| IBIS file stm32l0_51_52_53_62_63_tfbga64.ibs
| Created by s2ibis version 1.1 (customized version)
| North Carolina State University, ERL, 2006
[IBIS ver] 4.2
[File name] stm32l0_51_52_53_62_63_tfbga64.ibs
[File Rev] 1.0
[Date]  15-10-2014
[Source] Data Created at STMicroelectronics
[Notes]  File originated from ELDO simulations.
[Disclaimer]  This information is for modeling purpose only and is
   not guaranted. The information is subject to change without
   notice.
[Copyright] Copyright 2016 STMicroelectronics Inc.
|   Component stm32l0_51_52_53_62_63_tfbga64
[Component] stm32l0_51_52_53_62_63_tfbga64
[Manufacturer] STMicroelectronics
[Package]
| variable   typ   min   max
R_pkg   0.0   0.0   0.0
L_pkg   0.0H   0.0H   0.0H
C_pkg   0.0F   0.0F   0.0F
[Pin]  signal_name   model_name   R_pin   L_pin   C_pin
B2 VLCD POWER
A2 PC13 io8p_wsudq_ls_ft_v33
A1 PC14-OSC32_IN io8p_wsudq_ls_ft_v33
B1 PC15-OSC32_OUT io8p_sudq_ls_tc_esdft
C1 PH0-OSC_IN io8p_sudq_ls_tc_esdft
D1 PH1-OSC_OUT io8p_sudq_ls_tc_esdft
E1 NRST ioreset_tc_v33_esdft
E3 PC0 io8p_wsudq_lcd4_ls_ft
E2 PC1 io8p_wsudq_lcd4_ls_ft
F2 PC2 io8p_wsudq_lcd4_ls_ft
F1 VSSA GND
G1 VREF+ POWER
H1 VDDA POWER
G2 PA0 io8p_wsudq_ls_ft_v33
H2 PA1 io8p_wsudq_lcd4_ls_ft
F3 PA2 io8p_wsudq_lcd4_ls_ft
G3 PA3 io8p_wsudq_lcd4_ls_ft
C2 VSS GND
D2 VDD POWER
H3 PA4 io8p_wsudq_i2cin_ls_ft
F4 PA5 io8p_wsudq_i2cin_ls_ft
G4 PA6 io8p_wsudq_lcd4_ls_ft
H4 PA7 io8p_wsudq_lcd4_ls_ft
H5 PC4 io8p_wsudq_lcd4_ls_ft
H6 PC5 io8p_wsudq_lcd4_ls_ft
F5 PB0 io8p_wsudq_lcd4_ls_ft
G5 PB1 io8p_wsudq_lcd4_ls_ft
G6 PB2 io8p_wsudq_lcd4_ls_ft
G7 PB10 io8p_sudq_lcd4_i2cin_ls_ft
H7 PB11 io8p_sudq_lcd4_i2cin_ls_ft
D6 VSS GND
E5 VDD POWER
H8 PB12 io8p_wsudq_lcd4_ls_ft
G8 PB13 io8p_sudq_lcd4_i2cin_ls_ft
F8 PB14 io8p_sudq_lcd4_i2cin_ls_ft
F7 PB15 io8p_wsudq_lcd4_ls_ft
F6 PC6 io8p_wsudq_lcd4_ls_ft
E7 PC7 io8p_wsudq_lcd4_ls_ft
E8 PC8 io8p_wsudq_lcd4_ls_ft
D8 PC9 io8p_wsudq_lcd4_ls_ft
D7 PA8 io8p_wsudq_lcd4_ls_ft
C7 PA9 io8p_wsudq_lcd4_ls_ft
C6 PA10 io8p_wsudq_lcd4_ls_ft
C8 PA11 io8usb_ls_ft
B8 PA12 io8usb_ls_ft
A8 PA13 io8p_sudq_ls_ft
D5 VSS GND
E6 VDD_USB POWER
A7 PA14 io8p_sudq_ls_ft
A6 PA15 io8p_wsudq_lcd4_ls_ft
B7 PC10 io8p_wsudq_lcd4_ls_ft
B6 PC11 io8p_wsudq_lcd4_ls_ft
C5 PC12 io8p_wsudq_lcd4_ls_ft
B5 PD2 io8p_wsudq_lcd4_ls_ft
A5 PB3 io8p_wsudq_lcd4_ls_ft
A4 PB4 io8p_wsudq_lcd4_ls_ft
C4 PB5 io8p_wsudq_lcd4_ls_ft
D3 PB6 io8p_wsudq_i2cin_ls_ft
C3 PB7 io8p_wsudq_i2cin_ls_ft
B4 BOOT0 vpp_test_hv
B3 PB8 io8p_sudq_lcd4_i2cin_ls_ft
A3 PB9 io8p_sudq_lcd4_i2cin_ls_ft
D4 VSS_3 GND
E4 VDD_3 POWER
[Model Selector] io8p_sudq_ls_ft
io8p00_sudq_ls_ft_pd_lv  "SPEED00 1P8V, PD=40kOhm"
io8p00_sudq_ls_ft_pu_lv  "SPEED00 1P8V, PU=40kOhm"
io8p00_sudq_ls_ft_lv  "SPEED00 1P8V"
io8p01_sudq_ls_ft_pd_lv  "SPEED01 1P8V, PD=40kOhm"
io8p01_sudq_ls_ft_pu_lv  "SPEED01 1P8V, PU=40kOhm"
io8p01_sudq_ls_ft_lv  "SPEED01 1P8V"
io8p10_sudq_ls_ft_pd_lv  "SPEED10 1P8V, PD=40kOhm"
io8p10_sudq_ls_ft_pu_lv  "SPEED10 1P8V, PU=40kOhm"
io8p10_sudq_ls_ft_lv  "SPEED10 1P8V"
io8p11_sudq_ls_ft_pd_lv  "SPEED11 1P8V, PD=40kOhm"
io8p11_sudq_ls_ft_pu_lv  "SPEED11 1P8V, PU=40kOhm"
io8p11_sudq_ls_ft_lv  "SPEED11 1P8V"
io8p00_sudq_ls_ft_pd  "SPEED00, PD=40kOhm"
io8p00_sudq_ls_ft_pu  "SPEED00, PU=40kOhm"
io8p00_sudq_ls_ft  "SPEED00"
io8p01_sudq_ls_ft_pd  "SPEED01, PD=40kOhm"
io8p01_sudq_ls_ft_pu  "SPEED01, PU=40kOhm"
io8p01_sudq_ls_ft  "SPEED01"
io8p10_sudq_ls_ft_pd  "SPEED10, PD=40kOhm"
io8p10_sudq_ls_ft_pu  "SPEED10, PU=40kOhm"
io8p10_sudq_ls_ft  "SPEED10"
io8p11_sudq_ls_ft_pd  "SPEED11, PD=40kOhm"
io8p11_sudq_ls_ft_pu  "SPEED11, PU=40kOhm"
io8p11_sudq_ls_ft  "SPEED11"
[Model Selector] io8p_sudq_ls_tc_esdft
io8p00_sudq_ls_tc_esdft_pd_lv  "SPEED00 1P8V, PD=40kOhm"
io8p00_sudq_ls_tc_esdft_pu_lv  "SPEED00 1P8V, PU=40kOhm"
io8p00_sudq_ls_tc_esdft_lv  "SPEED00 1P8V"
io8p01_sudq_ls_tc_esdft_pd_lv  "SPEED01 1P8V, PD=40kOhm"
io8p01_sudq_ls_tc_esdft_pu_lv  "SPEED01 1P8V, PU=40kOhm"
io8p01_sudq_ls_tc_esdft_lv  "SPEED01 1P8V"
io8p10_sudq_ls_tc_esdft_pd_lv  "SPEED10 1P8V, PD=40kOhm"
io8p10_sudq_ls_tc_esdft_pu_lv  "SPEED10 1P8V, PU=40kOhm"
io8p10_sudq_ls_tc_esdft_lv  "SPEED10 1P8V"
io8p11_sudq_ls_tc_esdft_pd_lv  "SPEED11 1P8V, PD=40kOhm"
io8p11_sudq_ls_tc_esdft_pu_lv  "SPEED11 1P8V, PU=40kOhm"
io8p11_sudq_ls_tc_esdft_lv  "SPEED11 1P8V"
io8p00_sudq_ls_tc_esdft_pd  "SPEED00, PD=40kOhm"
io8p00_sudq_ls_tc_esdft_pu  "SPEED00, PU=40kOhm"
io8p00_sudq_ls_tc_esdft  "SPEED00"
io8p01_sudq_ls_tc_esdft_pd  "SPEED01, PD=40kOhm"
io8p01_sudq_ls_tc_esdft_pu  "SPEED01, PU=40kOhm"
io8p01_sudq_ls_tc_esdft  "SPEED01"
io8p10_sudq_ls_tc_esdft_pd  "SPEED10, PD=40kOhm"
io8p10_sudq_ls_tc_esdft_pu  "SPEED10, PU=40kOhm"
io8p10_sudq_ls_tc_esdft  "SPEED10"
io8p11_sudq_ls_tc_esdft_pd  "SPEED11, PD=40kOhm"
io8p11_sudq_ls_tc_esdft_pu  "SPEED11, PU=40kOhm"
io8p11_sudq_ls_tc_esdft  "SPEED11"
[Model Selector] io8p_wsudq_i2cin_ls_ft
io8p00_wsudq_i2cin_ls_ft_pd_lv  "SPEED00 1P8V, PD=40kOhm"
io8p00_wsudq_i2cin_ls_ft_pu_lv  "SPEED00 1P8V, PU=40kOhm"
io8p00_wsudq_i2cin_ls_ft_lv  "SPEED00 1P8V"
io8p01_wsudq_i2cin_ls_ft_pd_lv  "SPEED01 1P8V, PD=40kOhm"
io8p01_wsudq_i2cin_ls_ft_pu_lv  "SPEED01 1P8V, PU=40kOhm"
io8p01_wsudq_i2cin_ls_ft_lv  "SPEED01 1P8V"
io8p10_wsudq_i2cin_ls_ft_pd_lv  "SPEED10 1P8V, PD=40kOhm"
io8p10_wsudq_i2cin_ls_ft_pu_lv  "SPEED10 1P8V, PU=40kOhm"
io8p10_wsudq_i2cin_ls_ft_lv  "SPEED10 1P8V"
io8p11_wsudq_i2cin_ls_ft_pd_lv  "SPEED11 1P8V, PD=40kOhm"
io8p11_wsudq_i2cin_ls_ft_pu_lv  "SPEED11 1P8V, PU=40kOhm"
io8p11_wsudq_i2cin_ls_ft_lv  "SPEED11 1P8V"
io8p00_wsudq_i2cin_ls_ft_pd  "SPEED00, PD=40kOhm"
io8p00_wsudq_i2cin_ls_ft_pu  "SPEED00, PU=40kOhm"
io8p00_wsudq_i2cin_ls_ft  "SPEED00"
io8p01_wsudq_i2cin_ls_ft_pd  "SPEED01, PD=40kOhm"
io8p01_wsudq_i2cin_ls_ft_pu  "SPEED01, PU=40kOhm"
io8p01_wsudq_i2cin_ls_ft  "SPEED01"
io8p10_wsudq_i2cin_ls_ft_pd  "SPEED10, PD=40kOhm"
io8p10_wsudq_i2cin_ls_ft_pu  "SPEED10, PU=40kOhm"
io8p10_wsudq_i2cin_ls_ft  "SPEED10"
io8p11_wsudq_i2cin_ls_ft_pd  "SPEED11, PD=40kOhm"
io8p11_wsudq_i2cin_ls_ft_pu  "SPEED11, PU=40kOhm"
io8p11_wsudq_i2cin_ls_ft  "SPEED11"
[Model Selector] io8p_wsudq_lcd4_ls_ft
io8p00_wsudq_lcd4_ls_ft_pd_lv  "SPEED00 1P8V, PD=40kOhm"
io8p00_wsudq_lcd4_ls_ft_pu_lv  "SPEED00 1P8V, PU=40kOhm"
io8p00_wsudq_lcd4_ls_ft_lv  "SPEED00 1P8V"
io8p01_wsudq_lcd4_ls_ft_pd_lv  "SPEED01 1P8V, PD=40kOhm"
io8p01_wsudq_lcd4_ls_ft_pu_lv  "SPEED01 1P8V, PU=40kOhm"
io8p01_wsudq_lcd4_ls_ft_lv  "SPEED01 1P8V"
io8p10_wsudq_lcd4_ls_ft_pd_lv  "SPEED10 1P8V, PD=40kOhm"
io8p10_wsudq_lcd4_ls_ft_pu_lv  "SPEED10 1P8V, PU=40kOhm"
io8p10_wsudq_lcd4_ls_ft_lv  "SPEED10 1P8V"
io8p11_wsudq_lcd4_ls_ft_pd_lv  "SPEED11 1P8V, PD=40kOhm"
io8p11_wsudq_lcd4_ls_ft_pu_lv  "SPEED11 1P8V, PU=40kOhm"
io8p11_wsudq_lcd4_ls_ft_lv  "SPEED11 1P8V"
io8p00_wsudq_lcd4_ls_ft_pd  "SPEED00, PD=40kOhm"
io8p00_wsudq_lcd4_ls_ft_pu  "SPEED00, PU=40kOhm"
io8p00_wsudq_lcd4_ls_ft  "SPEED00"
io8p01_wsudq_lcd4_ls_ft_pd  "SPEED01, PD=40kOhm"
io8p01_wsudq_lcd4_ls_ft_pu  "SPEED01, PU=40kOhm"
io8p01_wsudq_lcd4_ls_ft  "SPEED01"
io8p10_wsudq_lcd4_ls_ft_pd  "SPEED10, PD=40kOhm"
io8p10_wsudq_lcd4_ls_ft_pu  "SPEED10, PU=40kOhm"
io8p10_wsudq_lcd4_ls_ft  "SPEED10"
io8p11_wsudq_lcd4_ls_ft_pd  "SPEED11, PD=40kOhm"
io8p11_wsudq_lcd4_ls_ft_pu  "SPEED11, PU=40kOhm"
io8p11_wsudq_lcd4_ls_ft  "SPEED11"
[Model Selector] io8p_wsudq_ls_ft_v33
io8p00_wsudq_ls_ft_v33_pd_lv  "SPEED00 1P8V, PD=40kOhm"
io8p00_wsudq_ls_ft_v33_pu_lv  "SPEED00 1P8V, PU=40kOhm"
io8p00_wsudq_ls_ft_v33_lv  "SPEED00 1P8V"
io8p01_wsudq_ls_ft_v33_pd_lv  "SPEED01 1P8V, PD=40kOhm"
io8p01_wsudq_ls_ft_v33_pu_lv  "SPEED01 1P8V, PU=40kOhm"
io8p01_wsudq_ls_ft_v33_lv  "SPEED01 1P8V"
io8p10_wsudq_ls_ft_v33_pd_lv  "SPEED10 1P8V, PD=40kOhm"
io8p10_wsudq_ls_ft_v33_pu_lv  "SPEED10 1P8V, PU=40kOhm"
io8p10_wsudq_ls_ft_v33_lv  "SPEED10 1P8V"
io8p11_wsudq_ls_ft_v33_pd_lv  "SPEED11 1P8V, PD=40kOhm"
io8p11_wsudq_ls_ft_v33_pu_lv  "SPEED11 1P8V, PU=40kOhm"
io8p11_wsudq_ls_ft_v33_lv  "SPEED11 1P8V"
io8p00_wsudq_ls_ft_v33_pd  "SPEED00, PD=40kOhm"
io8p00_wsudq_ls_ft_v33_pu  "SPEED00, PU=40kOhm"
io8p00_wsudq_ls_ft_v33  "SPEED00"
io8p01_wsudq_ls_ft_v33_pd  "SPEED01, PD=40kOhm"
io8p01_wsudq_ls_ft_v33_pu  "SPEED01, PU=40kOhm"
io8p01_wsudq_ls_ft_v33  "SPEED01"
io8p10_wsudq_ls_ft_v33_pd  "SPEED10, PD=40kOhm"
io8p10_wsudq_ls_ft_v33_pu  "SPEED10, PU=40kOhm"
io8p10_wsudq_ls_ft_v33  "SPEED10"
io8p11_wsudq_ls_ft_v33_pd  "SPEED11, PD=40kOhm"
io8p11_wsudq_ls_ft_v33_pu  "SPEED11, PU=40kOhm"
io8p11_wsudq_ls_ft_v33  "SPEED11"
[Model Selector] ioreset_tc_v33_esdft
ioreset_tc_v33_esdft_pu_lv  "IORESET 1P65V + PU=40kOhm"
ioreset_tc_v33_esdft_nopu_lv  "IORESET 1P65V"
ioreset_tc_v33_esdft_pu  "IORESET + PU=40kOhm"
ioreset_tc_v33_esdft_nopu  "IORESET"
[Model Selector] vpp_test_hv
vpp_test_hv_2p4  "Input Buffer 1P65V"
vpp_test_hv_3p3  "Input Buffer"
[Model Selector] io8usb_ls_ft
io8usb_ls_ft_dpdn_pu  "HS USB DP/DN IO + PU=1.2kOhm"
io8usb_ls_ft_dpdn  "HS USB DP/DN IO"
io8p00_ls_ft_pd_lv  "SPEED00 1P8V, PD=40kOhm"
io8p00_ls_ft_pu_lv  "SPEED00 1P8V, PU=40kOhm"
io8p00_ls_ft_lv  "SPEED00 1P8V"
io8p01_ls_ft_pd_lv  "SPEED01 1P8V, PD=40kOhm"
io8p01_ls_ft_pu_lv  "SPEED01 1P8V, PU=40kOhm"
io8p01_ls_ft_lv  "SPEED01 1P8V"
io8p10_ls_ft_pd_lv  "SPEED10 1P8V, PD=40kOhm"
io8p10_ls_ft_pu_lv  "SPEED10 1P8V, PU=40kOhm"
io8p10_ls_ft_lv  "SPEED10 1P8V"
io8p11_ls_ft_pd_lv  "SPEED11 1P8V, PD=40kOhm"
io8p11_ls_ft_pu_lv  "SPEED11 1P8V, PU=40kOhm"
io8p11_ls_ft_lv  "SPEED11 1P8V"
io8p00_ls_ft_pd  "SPEED00, PD=40kOhm"
io8p00_ls_ft_pu  "SPEED00, PU=40kOhm"
io8p00_ls_ft  "SPEED00"
io8p01_ls_ft_pd  "SPEED01, PD=40kOhm"
io8p01_ls_ft_pu  "SPEED01, PU=40kOhm"
io8p01_ls_ft  "SPEED01"
io8p10_ls_ft_pd  "SPEED10, PD=40kOhm"
io8p10_ls_ft_pu  "SPEED10, PU=40kOhm"
io8p10_ls_ft  "SPEED10"
io8p11_ls_ft_pd  "SPEED11, PD=40kOhm"
io8p11_ls_ft_pu  "SPEED11, PU=40kOhm"
io8p11_ls_ft  "SPEED11"
[Model Selector] io8p_sudq_lcd4_i2cin_ls_ft
io8p00_sudq_lcd4_i2cin_ls_ft_pd_lv  "SPEED00 1P8V, PD=40kOhm"
io8p00_sudq_lcd4_i2cin_ls_ft_pu_lv  "SPEED00 1P8V, PU=40kOhm"
io8p00_sudq_lcd4_i2cin_ls_ft_lv  "SPEED00 1P8V"
io8p01_sudq_lcd4_i2cin_ls_ft_pd_lv  "SPEED01 1P8V, PD=40kOhm"
io8p01_sudq_lcd4_i2cin_ls_ft_pu_lv  "SPEED01 1P8V, PU=40kOhm"
io8p01_sudq_lcd4_i2cin_ls_ft_lv  "SPEED01 1P8V"
io8p10_sudq_lcd4_i2cin_ls_ft_pd_lv  "SPEED10 1P8V, PD=40kOhm"
io8p10_sudq_lcd4_i2cin_ls_ft_pu_lv  "SPEED10 1P8V, PU=40kOhm"
io8p10_sudq_lcd4_i2cin_ls_ft_lv  "SPEED10 1P8V"
io8p11_sudq_lcd4_i2cin_ls_ft_pd_lv  "SPEED11 1P8V, PD=40kOhm"
io8p11_sudq_lcd4_i2cin_ls_ft_pu_lv  "SPEED11 1P8V, PU=40kOhm"
io8p11_sudq_lcd4_i2cin_ls_ft_lv  "SPEED11 1P8V"
io8p00_sudq_lcd4_i2cin_ls_ft_pd  "SPEED00, PD=40kOhm"
io8p00_sudq_lcd4_i2cin_ls_ft_pu  "SPEED00, PU=40kOhm"
io8p00_sudq_lcd4_i2cin_ls_ft  "SPEED00"
io8p01_sudq_lcd4_i2cin_ls_ft_pd  "SPEED01, PD=40kOhm"
io8p01_sudq_lcd4_i2cin_ls_ft_pu  "SPEED01, PU=40kOhm"
io8p01_sudq_lcd4_i2cin_ls_ft  "SPEED01"
io8p10_sudq_lcd4_i2cin_ls_ft_pd  "SPEED10, PD=40kOhm"
io8p10_sudq_lcd4_i2cin_ls_ft_pu  "SPEED10, PU=40kOhm"
io8p10_sudq_lcd4_i2cin_ls_ft  "SPEED10"
io8p11_sudq_lcd4_i2cin_ls_ft_pd  "SPEED11, PD=40kOhm"
io8p11_sudq_lcd4_i2cin_ls_ft_pu  "SPEED11, PU=40kOhm"
io8p11_sudq_lcd4_i2cin_ls_ft  "SPEED11"
| Models and submodels in the file (176): io8p00_sudq_ls_ft_pd_lv (I/O), io8p00_sudq_ls_ft_pu_lv (I/O), io8p00_sudq_ls_ft_lv (I/O), io8p01_sudq_ls_ft_pd_lv (I/O), io8p01_sudq_ls_ft_pu_lv (I/O), io8p01_sudq_ls_ft_lv (I/O), io8p10_sudq_ls_ft_pd_lv (I/O), io8p10_sudq_ls_ft_pu_lv (I/O), io8p10_sudq_ls_ft_lv (I/O), io8p11_sudq_ls_ft_pd_lv (I/O), io8p11_sudq_ls_ft_pu_lv (I/O), io8p11_sudq_ls_ft_lv (I/O), io8p00_sudq_ls_ft_pd (I/O), io8p00_sudq_ls_ft_pu (I/O), io8p00_sudq_ls_ft (I/O), io8p01_sudq_ls_ft_pd (I/O), io8p01_sudq_ls_ft_pu (I/O), io8p01_sudq_ls_ft (I/O), io8p10_sudq_ls_ft_pd (I/O), io8p10_sudq_ls_ft_pu (I/O), io8p10_sudq_ls_ft (I/O), io8p11_sudq_ls_ft_pd (I/O), io8p11_sudq_ls_ft_pu (I/O), io8p11_sudq_ls_ft (I/O), io8p00_sudq_ls_tc_esdft_pd_lv (I/O), io8p00_sudq_ls_tc_esdft_pu_lv (I/O), io8p00_sudq_ls_tc_esdft_lv (I/O), io8p01_sudq_ls_tc_esdft_pd_lv (I/O), io8p01_sudq_ls_tc_esdft_pu_lv (I/O), io8p01_sudq_ls_tc_esdft_lv (I/O), io8p10_sudq_ls_tc_esdft_pd_lv (I/O), io8p10_sudq_ls_tc_esdft_pu_lv (I/O), io8p10_sudq_ls_tc_esdft_lv (I/O), io8p11_sudq_ls_tc_esdft_pd_lv (I/O), io8p11_sudq_ls_tc_esdft_pu_lv (I/O), io8p11_sudq_ls_tc_esdft_lv (I/O), io8p00_sudq_ls_tc_esdft_pd (I/O), io8p00_sudq_ls_tc_esdft_pu (I/O), io8p00_sudq_ls_tc_esdft (I/O), io8p01_sudq_ls_tc_esdft_pd (I/O), io8p01_sudq_ls_tc_esdft_pu (I/O), io8p01_sudq_ls_tc_esdft (I/O), io8p10_sudq_ls_tc_esdft_pd (I/O), io8p10_sudq_ls_tc_esdft_pu (I/O), io8p10_sudq_ls_tc_esdft (I/O), io8p11_sudq_ls_tc_esdft_pd (I/O), io8p11_sudq_ls_tc_esdft_pu (I/O), io8p11_sudq_ls_tc_esdft (I/O), io8p00_wsudq_i2cin_ls_ft_pd_lv (I/O), io8p00_wsudq_i2cin_ls_ft_pu_lv (I/O), io8p00_wsudq_i2cin_ls_ft_lv (I/O), io8p01_wsudq_i2cin_ls_ft_pd_lv (I/O), io8p01_wsudq_i2cin_ls_ft_pu_lv (I/O), io8p01_wsudq_i2cin_ls_ft_lv (I/O), io8p10_wsudq_i2cin_ls_ft_pd_lv (I/O), io8p10_wsudq_i2cin_ls_ft_pu_lv (I/O), io8p10_wsudq_i2cin_ls_ft_lv (I/O), io8p11_wsudq_i2cin_ls_ft_pd_lv (I/O), io8p11_wsudq_i2cin_ls_ft_pu_lv (I/O), io8p11_wsudq_i2cin_ls_ft_lv (I/O), io8p00_wsudq_i2cin_ls_ft_pd (I/O), io8p00_wsudq_i2cin_ls_ft_pu (I/O), io8p00_wsudq_i2cin_ls_ft (I/O), io8p01_wsudq_i2cin_ls_ft_pd (I/O), io8p01_wsudq_i2cin_ls_ft_pu (I/O), io8p01_wsudq_i2cin_ls_ft (I/O), io8p10_wsudq_i2cin_ls_ft_pd (I/O), io8p10_wsudq_i2cin_ls_ft_pu (I/O), io8p10_wsudq_i2cin_ls_ft (I/O), io8p11_wsudq_i2cin_ls_ft_pd (I/O), io8p11_wsudq_i2cin_ls_ft_pu (I/O), io8p11_wsudq_i2cin_ls_ft (I/O), io8p00_wsudq_lcd4_ls_ft_pd_lv (I/O), io8p00_wsudq_lcd4_ls_ft_pu_lv (I/O), io8p00_wsudq_lcd4_ls_ft_lv (I/O), io8p01_wsudq_lcd4_ls_ft_pd_lv (I/O), io8p01_wsudq_lcd4_ls_ft_pu_lv (I/O), io8p01_wsudq_lcd4_ls_ft_lv (I/O), io8p10_wsudq_lcd4_ls_ft_pd_lv (I/O), io8p10_wsudq_lcd4_ls_ft_pu_lv (I/O)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
